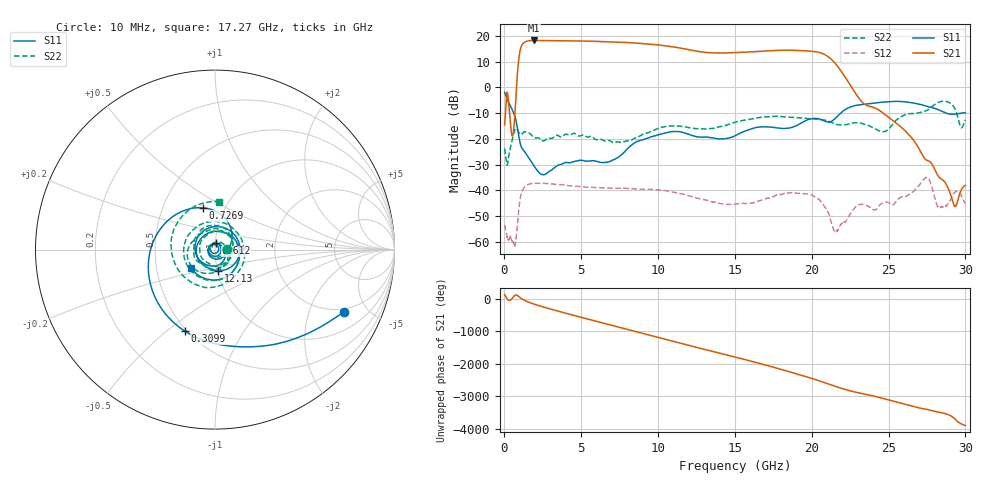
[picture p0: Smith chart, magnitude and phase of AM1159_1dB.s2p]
!Keysight Technologies,N5245B,MY58422270,A.16.20.02
!Date: Tuesday, December 10, 2024 22:56:31
!Correction: S11(C  2-Port  )
!S21(C  2-Port  )
!S12(C  2-Port  )
!S22(C  2-Port  )
!S2P File: Measurements: S11, S21, S12, S22:
# Hz S  dB  R 50
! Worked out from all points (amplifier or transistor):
!   6401 points, 10 MHz to 30 GHz, reference 50 ohm
!   highest |S21| = 18.2 dB at 1.894 GHz (marker M1)
!   |S21| within 3 dB of that: 1.055 GHz to 11.49 GHz (10.44 GHz wide, 166 % of centre)
!   unconditionally stable (mu >= 1): start of sweep to end of sweep
!   at 5.005 GHz: K = 5.31, MAG = 18.0 dB, |S12| = -38.5 dB
!   at 15.01 GHz: K = 18.72, MAG = 13.7 dB, |S12| = -45.4 dB
!   at 30 GHz: K = 6086.40, MAG = -37.4 dB, |S12| = -45.1 dB
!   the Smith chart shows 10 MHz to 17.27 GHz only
!   S11 on the Smith chart (normalised r, x): 10 MHz: 1.82, -3.45; 309.9 MHz: 0.49, -0.58; 726.9 MHz: 0.79, +0.39; 6.612 GHz: 1.01, +0.07; 12.13 GHz: 1.01, -0.24; 17.27 GHz: 0.75, -0.16
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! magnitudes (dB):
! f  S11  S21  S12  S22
! 10 MHz  -2.0  -14.6  -53.4  -23.8
! 183.4 MHz  -4.8  -1.9  -58.3  -30.2
! 309.9 MHz  -6.3  -8.7  -58.6  -25.6
! 525.5 MHz  -8.9  -18.9  -59.8  -19.7
! 726.9 MHz  -12.3  -5.7  -59.9  -16.0
! 1.083 GHz  -22.9  15.7  -41.4  -18.4
! 1.894 GHz  -30.3  18.2  -37.3  -19.4
! 2.554 GHz  -34.0  18.1  -37.3  -20.8
! 5.01 GHz  -28.3  18.0  -38.5  -18.7
! 6.612 GHz  -29.1  17.7  -39.0  -20.8
! 10.01 GHz  -18.5  16.4  -39.8  -16.0
! 12.13 GHz  -18.5  14.4  -42.3  -15.8
! 15.01 GHz  -18.8  13.4  -45.4  -13.6
! 17.27 GHz  -15.4  14.2  -42.9  -11.4
! 20 GHz  -12.2  13.9  -41.8  -12.2
! 21.56 GHz  -11.9  9.1  -56.1  -14.3
! 23 GHz  -6.9  -3.7  -45.8  -13.7
! 25 GHz  -5.6  -11.7  -44.8  -16.3
! 27.44 GHz  -7.3  -28.2  -35.0  -9.2
! 28.29 GHz  -8.9  -34.9  -46.8  -5.7
! 29.29 GHz  -10.4  -46.2  -40.8  -8.0
! 30 GHz  -9.9  -38.1  -45.1  -12.6
